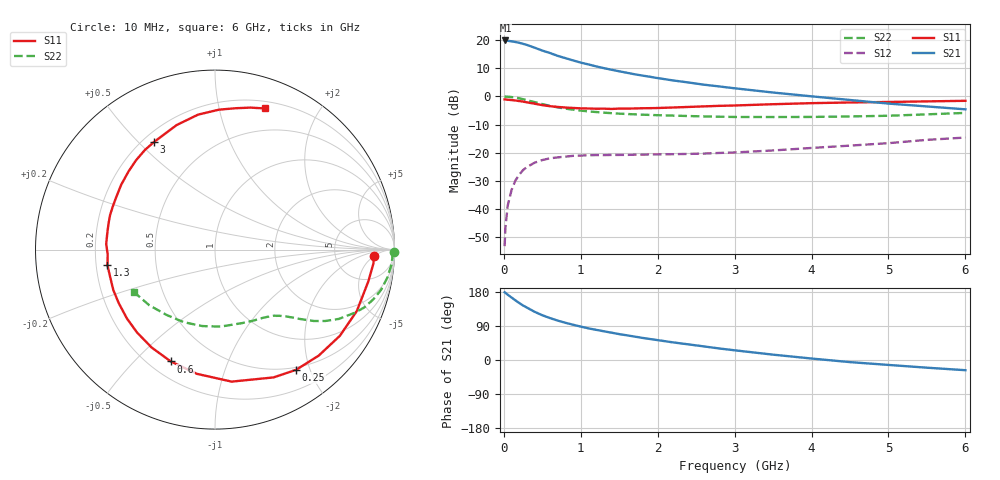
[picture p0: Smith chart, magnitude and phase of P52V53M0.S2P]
! SIEMENS Small Signal Semiconductors
! BFP183
! Si NPN RF Bipolar Junction Transistor in SOT143
! VCE = 2.5 V  IC = 3 mA
! Common Emitter S-Parameters:  March  1996
# GHz  S  MA  R  50
!  f  S11  S21  S12  S22
! GHz  MAG  ANG  MAG  ANG  MAG  ANG  MAG  ANG
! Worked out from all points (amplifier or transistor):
!   36 points, 10 MHz to 6 GHz, reference 50 ohm
!   highest |S21| = 19.8 dB at 20 MHz (marker M1)
!   |S21| within 3 dB of that: start of sweep to 442.3 MHz
!   unconditionally stable (mu >= 1): 1.87 GHz to 5.779 GHz
!   at 250 MHz: K = 0.15, MSG = 22.4 dB, |S12| = -26.1 dB
!   at 1.4 GHz: K = 0.80, MSG = 15.1 dB, |S12| = -20.8 dB
!   at 6 GHz: K = 0.96, MSG = 5.0 dB, |S12| = -14.6 dB
!   lowest NFmin = 1.10 dB at 450 MHz
!   S11 on the Smith chart (normalised r, x): 10 MHz: 15, -5; 250 MHz: 0.46, -1.79; 600 MHz: 0.28, -0.64; 1.3 GHz: 0.25, -0.07; 3 GHz: 0.24, +0.56; 6 GHz: 0.27, +1.38
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0.01  0.8838 -2.3  9.768 178.7  0.0022 85.2  0.9967 -0.9
0.02  0.8864 -4.9  9.821 177.4  0.0046 89.5  0.9899 -1.9
0.05  0.8725 -11.7  9.688 172.3  0.0115 86.3  0.9876 -4.7
0.1  0.8611 -23.4  9.487 164.9  0.0217 77.0  0.9726 -9.3
0.15  0.8455 -34.6  9.224 157.5  0.0321 70.5  0.9518 -13.7
0.2  0.8263 -45.6  8.933 150.5  0.0408 66.3  0.9242 -17.5
0.25  0.808 -56.0  8.553 143.8  0.0493 60.6  0.8917 -21.2
0.3  0.7832 -65.4  8.184 138.3  0.0557 56.0  0.8548 -24.3
0.4  0.7414 -82.8  7.307 127.2  0.0666 48.2  0.7913 -29.2
0.5  0.6996 -98.2  6.497 118.1  0.0742 41.7  0.7305 -33.0
0.6  0.67 -111.6  5.877 110.6  0.0798 36.8  0.6802 -35.8
0.7  0.6497 -122.9  5.236 104.0  0.0827 32.8  0.6381 -37.8
0.8  0.6341 -133.2  4.772 98.2  0.0853 29.5  0.6064 -39.5
1.1  0.6097 -158.4  3.689 83.5  0.0902 23.2  0.5412 -43.4
1.3  0.6055 -171.8  3.167 75.8  0.0908 20.9  0.514 -45.8
1.7  0.6107 166.4  2.466 61.8  0.0924 19.0  0.4803 -51.1
2.2  0.635 145.6  1.918 46.5  0.0943 19.4  0.4556 -58.7
3  0.6893 119.5  1.392 25.6  0.1012 22.6  0.4311 -74.5
3.5  0.7261 107.1  1.17 14.1  0.1098 24.4  0.4301 -85.8
4.5  0.7798 88.4  0.863 -5.6  0.1338 25.1  0.4404 -113.3
5.5  0.8153 76.0  0.663 -20.3  0.1693 22.6  0.4799 -139.8
6  0.834 70.6  0.589 -26.9  0.186 18.9  0.509 -152.1
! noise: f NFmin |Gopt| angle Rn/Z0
0.45  1.1  0.37  35  0.3
0.9  1.15  0.34  85  0.23
1.8  1.9  0.35  160  0.13
